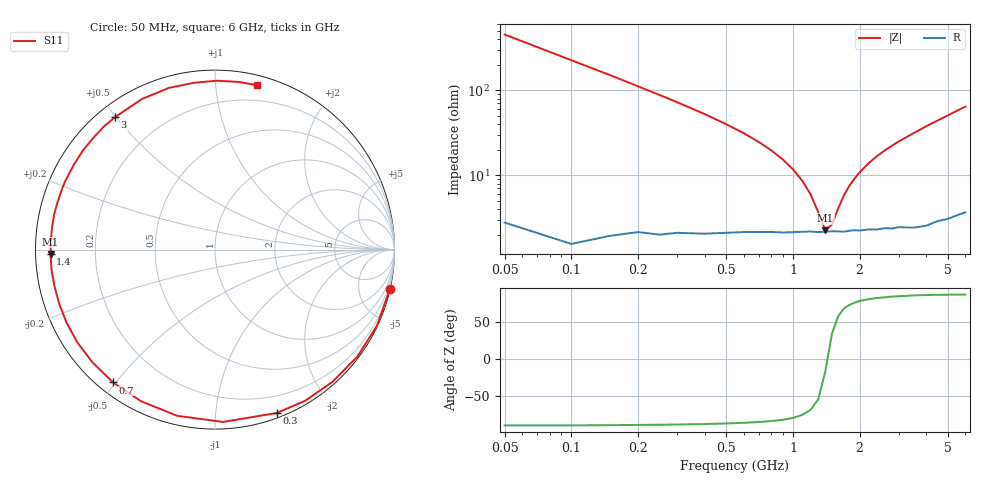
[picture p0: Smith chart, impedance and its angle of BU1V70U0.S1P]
! Infineon Technologies  Discrete & RF Semiconductors
! BB 833
! Si Tuning Diode in SOD323
! VR = 1.75 V
! S-Parameters:  June  1999
# GHz  S  MA  R  50
!  f  S11
! GHz  MAG  ANG
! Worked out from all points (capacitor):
!   34 points, 50 MHz to 6 GHz, reference 50 ohm
!   read as one part to ground: C = 7.02 pF near 50 MHz
!   lowest |Z| = 2.27 ohm at 1.4 GHz (marker M1)
!   series resonance near 1.431 GHz, so ESL is about 1.8 nH
!   S11 on the Smith chart (normalised r, x): 50 MHz: 0.06, -9.06; 300 MHz: 0.04, -1.45; 700 MHz: 0.04, -0.49; 1.4 GHz: 0.04, -0.01; 3 GHz: 0.05, +0.50; 6 GHz: 0.07, +1.28
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0.05  0.9987 -12.6
0.1  0.9971 -25.0
0.15  0.9923 -36.8
0.2  0.9857 -48.4
0.25  0.9807 -59.1
0.3  0.9732 -69.2
0.4  0.9615 -87.3
0.5  0.9497 -102.8
0.6  0.9399 -116.0
0.7  0.9329 -127.5
0.8  0.9278 -137.4
0.9  0.925 -146.1
1  0.9218 -153.9
1.1  0.919 -160.9
1.3  0.9177 -173.1
1.4  0.9168 -178.5
1.6  0.9164 172.1
1.8  0.9163 163.5
2  0.9177 156.0
2.4  0.9202 143.0
2.6  0.9204 137.2
3  0.9243 127.0
3.5  0.9325 116.0
4  0.9368 105.9
4.5  0.9369 97.1
5  0.941 89.3
5.5  0.9433 82.0
6  0.946 75.8
